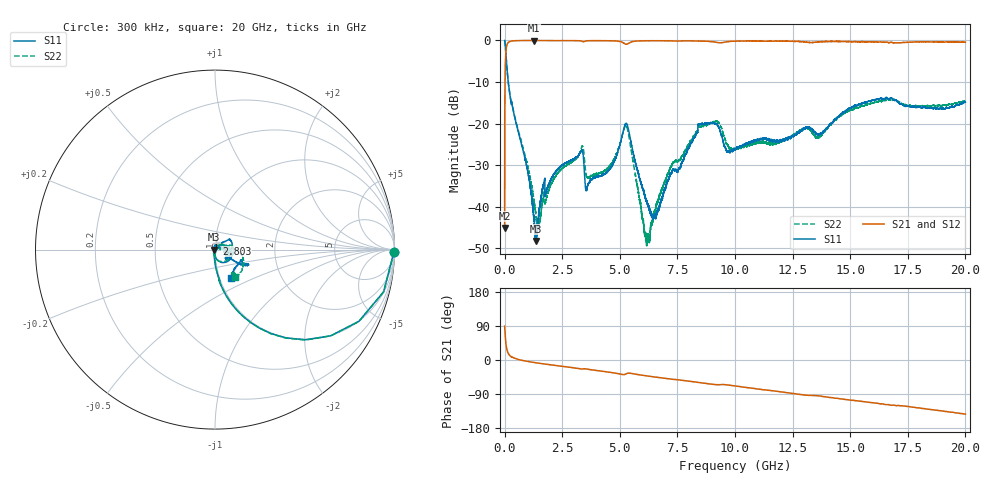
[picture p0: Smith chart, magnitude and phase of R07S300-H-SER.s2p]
!{R07S300}
!Johanson Technology Inc.
!www.johansontechnology.com
!Test Board Conditions:
!Substrate Type  RO4350B
!Substrate Thickness  10 mil
!Substrate Dk  3.66
!TL Type: GCPW
!TL Trace Width  21 mil
!TL Gap  20 mil
!Electrode orientation  Horizontal
!DUT TOPOLOGY	SERIES
!Mounting Pad LxW  16x21 mil
! Created Sat Feb  6 11:54:13 2021
# hz S ma R 50
! 2 Port Network Data from SP1.SP block
! freq  magS11  angS11  magS21  angS21  magS12  angS12  magS22  angS22
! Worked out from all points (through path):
!   20001 points, 300 kHz to 20 GHz, reference 50 ohm
!   highest |S21| = -0.01 dB at 1.29 GHz (marker M1); lowest = -45.1 dB at 300 kHz (marker M2)
!   group delay of S21, straight-line fit = 20.3 ps
!   lowest |S11| = -48.2 dB at 1.362 GHz (marker M3), VSWR 1.01, Z = 49.6 + j0.0176 ohm
!   |S11| at or under -10 dB: 158.5 MHz to end of sweep
!   |S22| runs from -49.5 to 0.0 dB; largest |S21 - S12| = 0.013
!   S11 on the Smith chart (normalised r, x): 300 kHz: open; 2.803 GHz: 1.01, +0.07; 20 GHz: 1.13, -0.37
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300000  0.9969 -0.7  0.005555 89.4  0.005583 87.7  0.9987 -0.7
1.013e8  0.4628 -63.2  0.8831 27.2  0.8838 27.1  0.4644 -63.1
1.423e8  0.3483 -70.8  0.9344 19.6  0.9357 19.6  0.3478 -70.8
1.0153e9  0.0257 -100.0  0.997 -4.0  0.9982 -4.0  0.02946 -89.3
1.2903e9  0.006386 -136.2  0.9983 -6.7  0.9961 -6.7  0.01083 -74.6
1.3623e9  0.003893 177.4  0.9974 -7.3  0.9969 -7.4  0.007695 -56.5
1.4833e9  0.008026 119.5  0.9968 -8.4  0.9973 -8.4  0.006018 -2.8
1.6493e9  0.01665 101.9  0.9966 -9.8  0.9963 -9.9  0.01152 39.2
2.8033e9  0.03526 78.5  0.9963 -19.1  0.995 -19.0  0.03309 51.6
3.3343e9  0.04735 55.1  0.9813 -23.7  0.982 -23.7  0.05086 36.4
3.6003e9  0.01791 62.0  0.9905 -24.2  0.9902 -24.2  0.02286 22.3
4.6323e9  0.03039 48.7  0.9901 -33.1  0.9904 -33.1  0.03286 43.0
5.2873e9  0.1002 -32.1  0.9001 -36.4  0.8994 -36.4  0.0927 -33.0
6.1373e9  0.01227 -72.4  0.991 -41.7  0.9913 -41.8  0.004152 164.9
6.6673e9  0.009111 11.0  0.9914 -46.0  0.992 -46.0  0.01178 53.4
8.4873e9  0.09792 36.0  0.9816 -59.8  0.9822 -59.8  0.09102 18.3
9.2403e9  0.09578 8.8  0.9449 -65.2  0.943 -65.2  0.1047 -11.4
9.6193e9  0.04824 0.9  0.9614 -65.4  0.9614 -65.3  0.05795 -24.0
1.00003e10  0.04967 10.5  0.9803 -68.6  0.9812 -68.6  0.04856 1.0
1.33343e10  0.08568 -38.3  0.9436 -93.4  0.9448 -93.5  0.07947 -25.9
1.66673e10  0.1977 -24.6  0.9399 -117.9  0.9459 -118.3  0.1939 -42.8
2e10  0.1813 -60.3  0.9522 -142.9  0.946 -142.8  0.1858 -54.5
